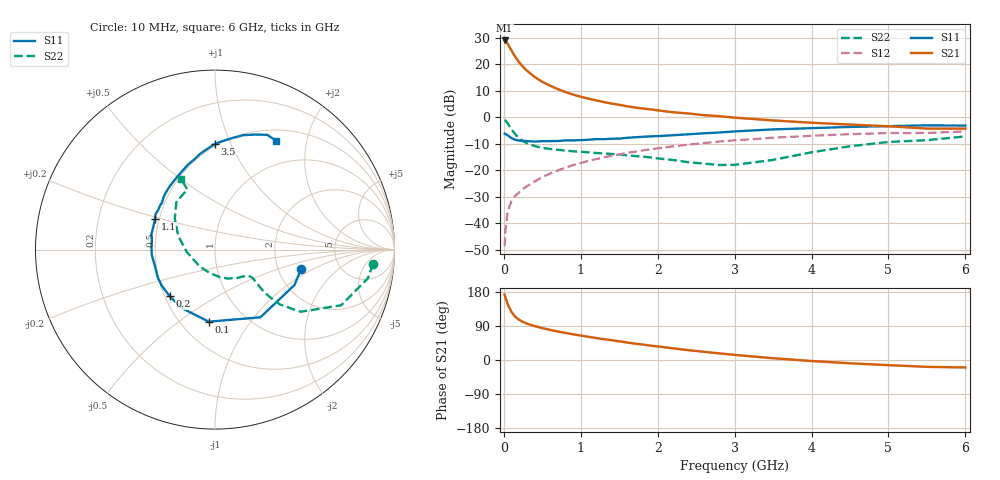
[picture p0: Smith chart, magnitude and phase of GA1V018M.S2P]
! Infineon Technologies  Discrete & RF Semiconductors
! BF775
! Si NPN RF Bipolar Junction Transistor in SOT23
! VCE = 1 V  IC = 18 mA
! Common Emitter S-Parameters:  May  1996
# GHz  S  MA  R  50
!  f  S11  S21  S12  S22
! GHz  MAG  ANG  MAG  ANG  MAG  ANG  MAG  ANG
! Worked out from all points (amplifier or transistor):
!   36 points, 10 MHz to 6 GHz, reference 50 ohm
!   highest |S21| = 29.0 dB at 10 MHz (marker M1)
!   |S21| within 3 dB of that: start of sweep to 83.68 MHz
!   unconditionally stable (mu >= 1): 228.4 MHz to end of sweep
!   at 250 MHz: K = 1.04, MAG = 21.8 dB, |S12| = -27.0 dB
!   at 1.4 GHz: K = 1.29, MAG = 6.6 dB, |S12| = -14.6 dB
!   at 6 GHz: K = 1.09, MAG = -1.3 dB, |S12| = -5.3 dB
!   S11 on the Smith chart (normalised r, x): 10 MHz: 2.70, -0.75; 100 MHz: 0.68, -0.65; 200 MHz: 0.53, -0.32; 1.1 GHz: 0.47, +0.19; 3.5 GHz: 0.48, +0.87; 6 GHz: 0.64, +1.51
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0.01  0.4926 -12.4  28.03 172.6  0.0037 83.1  0.8834 -5.2
0.02  0.4848 -24.0  27.48 165.5  0.0073 76.5  0.8671 -10.6
0.05  0.4542 -56.1  24.24 147.1  0.0168 69.6  0.7684 -23.8
0.1  0.4031 -94.9  18.01 126.5  0.0264 61.4  0.5894 -36.0
0.15  0.3745 -119.5  13.61 113.8  0.033 59.6  0.4736 -40.2
0.2  0.3622 -134.1  10.81 105.9  0.0384 60.6  0.3988 -40.9
0.25  0.3587 -145.9  8.903 100.3  0.0446 61.4  0.3526 -40.6
0.3  0.3546 -154.0  7.546 96.0  0.05 62.6  0.3247 -39.8
0.4  0.3473 -166.9  5.747 89.6  0.0614 64.5  0.286 -38.2
0.5  0.3534 -175.0  4.649 84.1  0.0741 65.9  0.2639 -37.1
0.6  0.3547 177.1  3.938 79.5  0.0865 66.2  0.2521 -37.1
0.8  0.3648 166.7  2.986 71.5  0.1117 65.7  0.2354 -38.6
0.9  0.3654 161.5  2.666 67.8  0.1249 65.1  0.2276 -39.8
1.1  0.3768 152.8  2.241 61.3  0.1499 63.6  0.2176 -43.7
1.3  0.3857 145.0  1.931 54.9  0.1752 61.4  0.2072 -48.0
1.6  0.4087 134.6  1.609 46.2  0.2119 57.7  0.1917 -56.4
2.2  0.4574 117.4  1.241 30.8  0.2821 49.6  0.1562 -79.8
2.8  0.5151 103.0  1.048 17.6  0.3471 40.8  0.1257 -119.4
3.5  0.5895 90.1  0.87 4.7  0.4102 30.1  0.1568 -174.9
4.5  0.6563 76.2  0.727 -8.7  0.4788 15.6  0.2833 142.3
5.5  0.7027 65.5  0.61 -18.1  0.5053 1.7  0.3691 114.7
6  0.695 60.8  0.611 -19.7  0.5404 -2.3  0.4348 115.7
